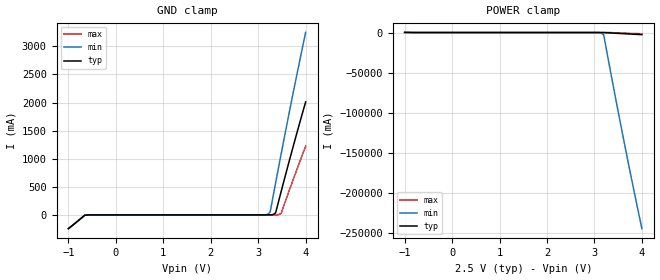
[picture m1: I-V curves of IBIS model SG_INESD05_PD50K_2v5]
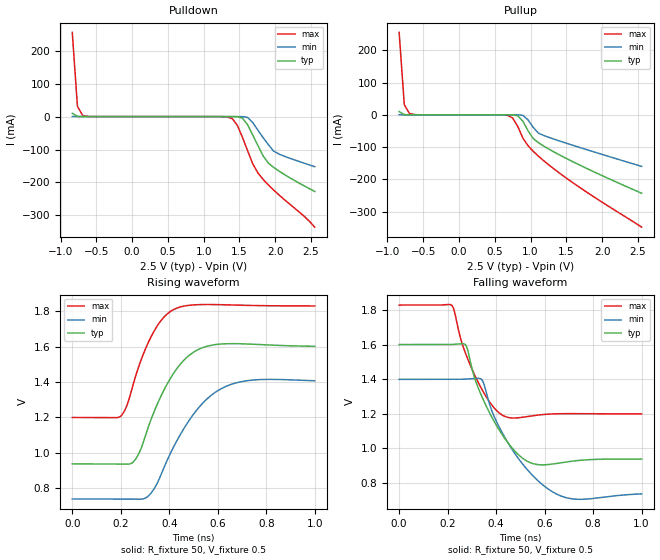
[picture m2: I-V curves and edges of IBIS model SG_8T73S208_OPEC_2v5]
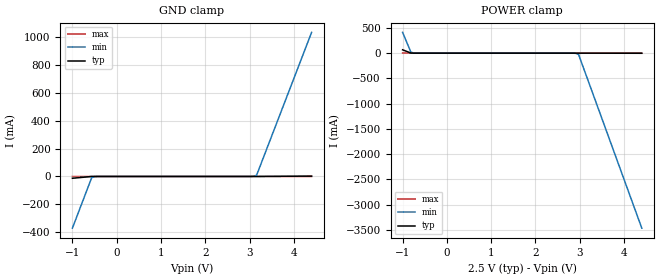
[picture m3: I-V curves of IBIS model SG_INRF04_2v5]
|   This file is an IBIS representation of the   |
|   Integrated Device Technology Inc   |
|   IDT8T732S208I-01   |
|   2.5V DIFFERENTIAL LVPECL CLOCK DIVIDER AND FANOUT BUFFER   |
[IBIS Ver]   4.1
[File name]   8t73s208i_01.ibs
[File Rev]   1.0
[Date]   14 APR 2015
[Source]   Originated at Integrated Device Technology, Inc.
[Disclaimer]
IDT hereby grants the user of this IBIS model a non-exclusive,
nontransferable license to use this IBIS model under the following terms.
Before using this IBIS model, the user should read this license.
If the user does not accept these terms,  the IBIS model should be
returned to IDT within 30 days.
   The user is granted this license only to use the IBIS model and
is not granted rights to sell, load, rent, lease or license the IBIS
model in whole or in part, or in modified form to anyone other than
user. User may modify the IBIS model to suit its specific
applications but rights to derivative works and such modifications
shall belong to IDT.
   This IBIS model is provided on an "AS IS" basis and IDT makes
absolutely no warranty with respect to the information contained
herein. IDT DISCLAIMS AND CUSTOMER WAIVES ALL WARRANTIES, EXPRESS
OR IMPLIED, INCLUDING WARRANTIES OF MERCHANTABILITY OR FITNESS FOR
A PARTICULAR PURPOSE. The entire risk as to quality and performance
is with the Customer. ACCORDINGLY, IN NO EVENT SHALL THE COMPANY BE
LIABLE FOR ANY DAMAGES, WHETHER IN CONTRACT OR TORT,INCLUDING ANY
LOST PROFITS OR OTHER INCIDENTAL, CONSEQUENTIAL, EXEMPLARY, OR
PUNITIVE DAMAGES ARISING OUT OF THE USE OR APPLICATION OF THE IBIS
model provided in this package. Further, IDT reserves the right to
make changes without notice to any product herein to improve
reliability, function, or design. IDT does not convey any license
under patent rights or any other intellectual property rights,
including those of third parties.
   IDT is not obligated to provide maintenance or support
for the licensed IBIS model.
[Copyright]   Copyright 2015 by IDT Inc.
[Component]   IDT8T73S208-01NGLI
[Manufacturer] Integrated Device Technology, Inc.
[Package]
|QFN 32
|lead + wire   typ   min   max
R_pkg   148.525m   92.309m   189.241m
L_pkg   1.318n   1.032n   1.634n
C_pkg   203.71f   184.14f   234.70f
[Pin] signal_name  model_name   R_pin   L_pin   C_pin
1   ADR1   SG_INESD05_PD50K   179.610m   1.461n   191.255f
2   VEE   GND   161.763m   1.447n   217.440f
3   Q0   SG_8T73S208_OPEC   133.456m   1.141n   193.994f
4   nQ0   SG_8T73S208_OPEC   121.044m   1.074n   185.939f
5   Q1   SG_8T73S208_OPEC   121.059m   1.076n   185.852f
6   nQ1   SG_8T73S208_OPEC   133.102m   1.147n   191.453f
7   VEE   GND   155.227m   1.389n   208.655f
8   VCCO   POWER   92.957m   1.034n   234.700f
9   Q2   SG_8T73S208_OPEC   189.241m   1.628n   200.299f
10   nQ2   SG_8T73S208_OPEC   162.649m   1.454n   218.396f
11   Q3   SG_8T73S208_OPEC   148.929m   1.333n   206.721f
12   nQ3   SG_8T73S208_OPEC   141.884m   1.269n   201.683f
13   Q4   SG_8T73S208_OPEC   140.676m   1.266n   201.115f
14   nQ4   SG_8T73S208_OPEC   147.702m   1.330n   206.004f
15   Q5   SG_8T73S208_OPEC   162.346m   1.447n   217.794f
16   nQ5   SG_8T73S208_OPEC   187.699m   1.617n   199.589f
17   VCCO   POWER   92.309m   1.032n   233.375f
18   VEE   GND   160.583m   1.439n   216.539f
19   Q6   SG_8T73S208_OPEC   130.493m   1.132n   190.219f
20   nQ6   SG_8T73S208_OPEC   119.346m   1.058n   184.145f
21   Q7   SG_8T73S208_OPEC   119.470m   1.058n   184.836f
22   nQ7   SG_8T73S208_OPEC   131.938m   1.123n   192.881f
23   VEE   GND   154.094m   1.380n   207.790f
24   FSEL0   SG_INESD05_PD50K   178.400m   1.450n   190.311f
25   FSEL1   SG_INESD05_PD50K   188.238m   1.619n   199.880f
26   IN   SG_INRF04   162.205m   1.453n   218.726f
27   VT   NC   148.673m   1.335n   206.818f
28   nIN   SG_INRF04   142.492m   1.275n   201.850f
29   VCC   POWER   143.017m   1.278n   202.447f
30   SDA   SG_I2C_DATAOUT02   149.682m   1.341n   207.211f
31   SCL   SG_I2C_SCLOCK03   163.397m   1.462n   219.637f
32   ADR0   SG_INESD05_PD50K   189.125m   1.634n   201.172f
[Diff Pin]  inv_pin   vdiff   tdelay_typ   tdelay_min   tdelay_max
3   4   NA   0   0   0
5   6   NA   0   0   0
9   10   NA   0   0   0
11   12   NA   0   0   0
13   14   NA   0   0   0
15   16   NA   0   0   0
19   20   NA   0   0   0
21   22   NA   0   0   0
26   28   0.15   NA   NA   NA
[Series Pin Mapping] Pin_2   model_name   function_table_group
26   28   ODT_100
[Model Selector] SG_INESD05_PD50K
SG_INESD05_PD50K_2v5  Buffer selection for 2v5
SG_INESD05_PD50K_3v3  Buffer selection for 3v3
[Model Selector] SG_8T73S208_OPEC
SG_8T73S208_OPEC_2v5  Buffer selection for 2v5
SG_8T73S208_OPEC_3v3  Buffer selection for 3v3
[Model Selector] SG_INRF04
SG_INRF04_2v5  Buffer selection for 2v5
SG_INRF04_3v3  Buffer selection for 3v3
[Model Selector] SG_I2C_DATAOUT02
SG_I2C_DATAOUT02_2v5  Buffer selection for 2v5
SG_I2C_DATAOUT02_3v3  Buffer selection for 3v3
[Model Selector] SG_I2C_SCLOCK03
SG_I2C_SCLOCK03_2v5  Buffer selection for 2v5
SG_I2C_SCLOCK03_3v3  Buffer selection for 3v3
[Model]   ODT_100
Model_type  Series
Polarity   Non-Inverting
|   typ   min   max
C_comp   0pF   0pF   0pF
|   typ   min   max
[Voltage Range]   3.3V   3.135V   3.465V
[R Series]   100ohm   80ohm   120ohm
| Models and submodels in the file (11): ODT_100 (Series), SG_INESD05_PD50K_2v5 (Input), SG_8T73S208_OPEC_2v5 (Output_ECL), SG_INRF04_2v5 (Input), SG_I2C_DATAOUT02_2v5 (Input), SG_I2C_SCLOCK03_2v5 (Input), SG_INESD05_PD50K_3v3 (Input), SG_8T73S208_OPEC_3v3 (Output_ECL), SG_INRF04_3v3 (Input), SG_I2C_DATAOUT02_3v3 (Input), SG_I2C_SCLOCK03_3v3 (Input)
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[Model] SG_INESD05_PD50K_2v5
Model_type   Input
Polarity   Non-Inverting
Vinl = 0.7V
Vinh = 1.7V
|   typ   min   max
C_comp   2pF   1.5pF   2.5pF
|   typ   min   max
[Voltage range]   2.5V   2.375V   2.625V
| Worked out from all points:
|   GND clamp passes 1 mA (typ) near -0.58 V on its own axis
|   POWER clamp passes 1 mA (typ) near -0.76 V on its own axis
[GND_clamp]
|Voltage   I (typ)   I (min)   I (max)
-999mV    -244.8mA   -244.8mA   -244.8mA
-654.2mV  -6.145mA   -6.145mA   -6.145mA
-596.8mV  -1.247mA   -1.247mA   -1.247mA
3.196V    197uA      6.481mA    69.73uA
3.253V    701.9uA    51.67mA    91.7uA
3.31V     4.516mA    312.6mA    170.5uA
3.368V    36.44mA    571mA      537.5uA
3.483V    411.8mA    1.08A      25.29mA
3.713V    1.14A      2.068A     570.6mA
4V        2.011A     3.248A     1.222A
[Power_clamp]
|Voltage   I (typ)   I (min)   I (max)
-999mV    170.5mA    170.5mA    170.5mA
3.081V    -874.7uA   -37.46mA   -65.82uA
3.138V    -3.712mA   -330.8mA   -230uA
3.196V    -25.84mA   -3.028A    -710.8uA
3.368V    -616.5mA   -57.72A    -152.9mA
3.598V    -1.377A    -128.1A    -679.2mA
3.77V     -1.927A    -179.1A    -1.06A
4V        -2.636A    -244.7A    -1.551A
[Model] SG_8T73S208_OPEC_2v5
Model_type   Output_ECL
Polarity   Non-Inverting
|   typ   min   max
C_comp   2pF   1.5pF   2.5pF
Vmeas = 1.27V
Rref = 50
Cref = 0
Vref = 0.5V
|   typ   min   max
[Voltage range]   2.5V   2.375V   2.625V
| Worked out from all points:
|   rising waveform, R_fixture 50, V_fixture 0.5: 20-80 % time 132ps typ, 168ps min, 105ps max; typ from 0.935 V to 1.6 V
|   falling waveform, R_fixture 50, V_fixture 0.5: 20-80 % time 130ps typ, 163ps min, 106ps max; typ from 1.6 V to 0.936 V
[Pulldown]
|Voltage   I (typ)   I (min)   I (max)
|Note, modeling breaks down at 250mA and above.  This is well beyond the functional   |
|operating range of the device.  Should this scenario occur, catastrophic failure and   |
|possible damage to the device and/or board is of higher concern than the I-V curve   |
|behavior.  The IBIS checker will flag currents in excess of 10A with warnings.  Lines   |
|with currents in excess of 0.35 A have been commented out.  The points still remain|
|available to the user if the user desires to use them.   |
|-2.40000e+00   2.40058e+08   3.18314e+08   1.70330e+08
|-2.30000e+00   2.17517e+08   2.89489e+08   1.53450e+08
|-2.20000e+00   1.94976e+08   2.60664e+08   1.36571e+08
|-2.10000e+00   1.72434e+08   2.31839e+08   1.19691e+08
|-2.00000e+00   1.49893e+08   2.03013e+08   1.02811e+08
|-1.99000e+00   1.47639e+08   2.00131e+08   1.01123e+08
|-1.91789e+00   1.31385e+08   1.79344e+08   8.89513e+07
|-1.84578e+00   1.15130e+08   1.58558e+08   7.67792e+07
|-1.77367e+00   9.88755e+07   1.37772e+08   6.46072e+07
|-1.70156e+00   8.26209e+07   1.16986e+08   5.24351e+07
|-1.62944e+00   6.63663e+07   9.61996e+07   4.02630e+07
|-1.55733e+00   5.01117e+07   7.54133e+07   2.80910e+07
|-1.48522e+00   3.38571e+07   5.46271e+07   1.59189e+07
|-1.41311e+00   1.76025e+07   3.38409e+07   4.06873e+06
|-1.34100e+00   2.68882e+06   1.30547e+07   4.97358e+05
|-1.26889e+00   1.62424e+05   5.60643e+05   6.08111e+04
|-1.19678e+00   9.82536e+03   1.55006e+04   7.44651e+03
|-1.12467e+00   6.03162e+02   4.37674e+02   9.19844e+02
|-1.05256e+00   4.08696e+01   1.46783e+01   1.18373e+02
|-9.80444e-01   2.72626e+00   4.11433e-01   1.67167e+01
|-9.08333e-01   1.64665e-01   1.13631e-02   2.09236e+00
-836.2mV  9.946mA    313.8uA    255.8mA
-764.1mV  600.7uA    8.668uA    31.26mA
-692mV    36.28uA    239.4nA    3.821mA
1.399V    -23.93uA   -81.46nA   -6.063mA
1.471V    -371.6uA   -2.797uA   -26.61mA
1.543V    -4.74mA    -95.28uA   -63.33mA
1.616V    -25.22mA   -2.607mA   -104.3mA
1.688V    -56.51mA   -18.58mA   -143.8mA
1.76V     -88.62mA   -41.74mA   -171.4mA
1.832V    -119.4mA   -64.05mA   -190.7mA
1.976V    -153.8mA   -104.3mA   -222.5mA
2.553V    -227.4mA   -152mA     -335.5mA
| 2.62511e+00   -2.35788e-01   -1.57199e-01   -3.55079e-01
| 2.69722e+00   -2.44484e-01   -1.62478e-01   -3.76294e-01
| 2.76933e+00   -2.54060e-01   -1.67881e-01   -3.98352e-01
| 2.84144e+00   -2.64769e-01   -1.73383e-01   -4.20357e-01
| 2.91356e+00   -2.76399e-01   -1.79146e-01   -4.42244e-01
| 2.98567e+00   -2.88756e-01   -1.85542e-01   -4.64335e-01
| 3.05778e+00   -3.01671e-01   -1.92630e-01   -4.83732e-01
| 3.12989e+00   -3.14773e-01   -2.00258e-01   -5.01249e-01
| 3.20200e+00   -3.28189e-01   -2.08432e-01   -5.18585e-01
| 3.27411e+00   -3.42273e-01   -2.18697e-01   -5.37304e-01
| 3.34622e+00   -3.64261e-01   -2.55817e-01   -5.66211e-01
| 3.41833e+00   -4.09420e-01   -3.05414e-01   -6.08363e-01
| 3.49044e+00   -4.54655e-01   -3.54748e-01   -6.50575e-01
| 3.56256e+00   -4.99420e-01   -4.03513e-01   -6.92819e-01
| 3.63467e+00   -5.44118e-01   -4.52081e-01   -7.35068e-01
| 3.70678e+00   -5.88861e-01   -5.00706e-01   -7.77241e-01
| 3.77889e+00   -6.33554e-01   -5.49415e-01   -8.19100e-01
| 3.85100e+00   -6.78004e-01   -5.98203e-01   -8.60639e-01
| 3.92311e+00   -7.21963e-01   -6.47066e-01   -9.01982e-01
| 3.99522e+00   -7.65389e-01   -6.95996e-01   -9.43201e-01
| 4.06733e+00   -8.08562e-01   -7.44993e-01   -9.84333e-01
| 4.13944e+00   -8.51732e-01   -7.94061e-01   -1.02539e+00
| 4.21156e+00   -8.94966e-01   -8.43201e-01   -1.06639e+00
| 4.28367e+00   -9.38253e-01   -8.92407e-01   -1.10739e+00
| 4.35578e+00   -9.81577e-01   -9.41676e-01   -1.14879e+00
| 4.42789e+00   -1.02499e+00   -9.91033e-01   -1.19324e+00
| 4.50000e+00   -1.06928e+00   -1.04102e+00   -1.23986e+00
| 4.51000e+00   -1.07571e+00   -1.04813e+00   -1.24627e+00
| 4.60800e+00   -1.14301e+00   -1.12225e+00   -1.30851e+00
| 4.70600e+00   -1.21072e+00   -1.19824e+00   -1.37003e+00
| 4.80400e+00   -1.27948e+00   -1.27431e+00   -1.43183e+00
| 4.90200e+00   -1.35101e+00   -1.35037e+00   -1.49633e+00
| 5.00000e+00   -1.42381e+00   -1.42638e+00   -1.56424e+00
[Pullup]
|Voltage   I (typ)   I (min)   I (max)
|Note, modeling breaks down at 250mA and above.  This is well beyond the functional   |
|operating range of the device.  Should this scenario occur, catastrophic failure and   |
|possible damage to the device and/or board is of higher concern than the I-V curve   |
|behavior.  The IBIS checker will flag currents in excess of 10A with warnings.  Lines   |
|with currents in excess of 0.35 A have been commented out.  The points still remain|
|available to the user if the user desires to use them.   |
|-2.40000e+00   2.40058e+08   3.18314e+08   1.70330e+08
|-2.30000e+00   2.17517e+08   2.89489e+08   1.53450e+08
|-2.20000e+00   1.94976e+08   2.60664e+08   1.36571e+08
|-2.10000e+00   1.72434e+08   2.31839e+08   1.19691e+08
|-2.00000e+00   1.49893e+08   2.03013e+08   1.02811e+08
|-1.99000e+00   1.47639e+08   2.00131e+08   1.01123e+08
|-1.91789e+00   1.31385e+08   1.79344e+08   8.89513e+07
|-1.84578e+00   1.15130e+08   1.58558e+08   7.67792e+07
|-1.77367e+00   9.88755e+07   1.37772e+08   6.46072e+07
|-1.70156e+00   8.26209e+07   1.16986e+08   5.24351e+07
|-1.62944e+00   6.63663e+07   9.61996e+07   4.02630e+07
|-1.55733e+00   5.01117e+07   7.54133e+07   2.80910e+07
|-1.48522e+00   3.38571e+07   5.46271e+07   1.59189e+07
|-1.41311e+00   1.76025e+07   3.38409e+07   4.06873e+06
|-1.34100e+00   2.68882e+06   1.30547e+07   4.97358e+05
|-1.26889e+00   1.62424e+05   5.60643e+05   6.08111e+04
|-1.19678e+00   9.82536e+03   1.55006e+04   7.44651e+03
|-1.12467e+00   6.03162e+02   4.37674e+02   9.19844e+02
|-1.05256e+00   4.08696e+01   1.46783e+01   1.18373e+02
|-9.80444e-01   2.72626e+00   4.11433e-01   1.67167e+01
|-9.08333e-01   1.64665e-01   1.13631e-02   2.09236e+00
-836.2mV  9.946mA    313.8uA    255.8mA
-764.1mV  600.7uA    8.668uA    31.26mA
-692mV    36.28uA    239.4nA    3.821mA
678.1mV   -14.48uA   -54.93nA   -1.577mA
750.2mV   -226.4uA   -1.885uA   -9.926mA
822.3mV   -3.108mA   -64.41uA   -36.27mA
894.4mV   -20.23mA   -1.876mA   -72.78mA
1.039V    -73.94mA   -39.15mA   -113.4mA
1.111V    -86.46mA   -56.96mA   -128.4mA
1.183V    -96.82mA   -63.97mA   -142.2mA
1.688V    -155.9mA   -101.3mA   -225.3mA
2.553V    -243.3mA   -160mA     -348.5mA
| 2.62511e+00   -2.50387e-01   -1.64771e-01   -3.59518e-01
| 2.69722e+00   -2.57594e-01   -1.69555e-01   -3.72316e-01
| 2.76933e+00   -2.64885e-01   -1.74366e-01   -3.87671e-01
| 2.84144e+00   -2.72208e-01   -1.79242e-01   -4.05741e-01
| 2.91356e+00   -2.79574e-01   -1.84271e-01   -4.25992e-01
| 2.98567e+00   -2.87321e-01   -1.89722e-01   -4.47114e-01
| 3.05778e+00   -2.96533e-01   -1.95679e-01   -4.68617e-01
| 3.12989e+00   -3.07573e-01   -2.02058e-01   -4.90289e-01
| 3.20200e+00   -3.19975e-01   -2.08904e-01   -5.11805e-01
| 3.27411e+00   -3.34016e-01   -2.18132e-01   -5.33959e-01
| 3.34622e+00   -3.56179e-01   -2.54416e-01   -5.65575e-01
| 3.41833e+00   -4.02130e-01   -3.03378e-01   -6.09689e-01
| 3.49044e+00   -4.48787e-01   -3.52496e-01   -6.52787e-01
| 3.56256e+00   -4.95341e-01   -4.01686e-01   -6.95001e-01
| 3.63467e+00   -5.41211e-01   -4.50852e-01   -7.36639e-01
| 3.70678e+00   -5.85960e-01   -4.99624e-01   -7.77908e-01
| 3.77889e+00   -6.30161e-01   -5.48368e-01   -8.18937e-01
| 3.85100e+00   -6.74093e-01   -5.97153e-01   -8.59793e-01
| 3.92311e+00   -7.17871e-01   -6.45989e-01   -9.00510e-01
| 3.99522e+00   -7.61550e-01   -6.94878e-01   -9.41084e-01
| 4.06733e+00   -8.05163e-01   -7.43823e-01   -9.81499e-01
| 4.13944e+00   -8.48736e-01   -7.92832e-01   -1.02174e+00
| 4.21156e+00   -8.92288e-01   -8.41909e-01   -1.06180e+00
| 4.28367e+00   -9.35825e-01   -8.91049e-01   -1.10177e+00
| 4.35578e+00   -9.79351e-01   -9.40247e-01   -1.14226e+00
| 4.42789e+00   -1.02293e+00   -9.89545e-01   -1.18633e+00
| 4.50000e+00   -1.06742e+00   -1.03964e+00   -1.23277e+00
| 4.51000e+00   -1.07388e+00   -1.04679e+00   -1.23919e+00
| 4.60800e+00   -1.14138e+00   -1.12122e+00   -1.30175e+00
| 4.70600e+00   -1.20927e+00   -1.19727e+00   -1.36399e+00
| 4.80400e+00   -1.27873e+00   -1.27338e+00   -1.42722e+00
| 4.90200e+00   -1.35081e+00   -1.34953e+00   -1.49362e+00
| 5.00000e+00   -1.42383e+00   -1.42570e+00   -1.56248e+00
[Ramp]
|   typ   min   max
dV/dt_r   0.409/0.137n   0.407/0.172n   0.384/0.108n
dV/dt_f   0.421/0.142n   0.421/0.178n   0.395/0.113n
R_load =   50.0000
[Rising Waveform]
R_fixture = 50
V_fixture = 0.5   | VCC_typ - 2V
V_fixture_max = 0.625   | VCC_max - 2V
V_fixture_min = 0.375   | VCC_min - 2V
C_fixture = 0.0p
| Time   typ   min   max
0s        935.3mV    736.8mV    1.198V
195.2ps   934.5mV    736.6mV    1.202V
223.2ps   933.5mV    736.5mV    1.259V
250.2ps   944.8mV    735.6mV    1.381V
281.3ps   1.014V     735.3mV    1.515V
327.3ps   1.196V     774.6mV    1.662V
423.4ps   1.46V      1.046V     1.813V
526.5ps   1.588V     1.262V     1.838V
630.6ps   1.616V     1.373V     1.836V
1ns       1.601V     1.406V     1.83V
[Falling Waveform]
R_fixture = 50
V_fixture = 0.5   | VCC_typ - 2V
V_fixture_max = 0.625   | VCC_max - 2V
V_fixture_min = 0.375   | VCC_min - 2V
C_fixture = 0.0p
| Time   typ   min   max
0s        1.601V     1.399V     1.83V
216.2ps   1.601V     1.399V     1.829V
272.3ps   1.601V     1.4V       1.555V
342.3ps   1.295V     1.394V     1.338V
384.4ps   1.174V     1.208V     1.246V
433.4ps   1.06V      1.068V     1.185V
536.5ps   917.8mV    861.8mV    1.185V
662.7ps   913.8mV    724.5mV    1.199V
752.8ps   929.7mV    702.7mV    1.2V
1ns       935.9mV    734.2mV    1.198V
[Model] SG_INRF04_2v5
Model_type   Input
Polarity   Non-Inverting
Vinl = 0.7V
Vinh = 1.7V
|   typ   min   max
C_comp   2pF   1.5pF   2.5pF
|   typ   min   max
[Voltage range]   2.5V   2.375V   2.625V
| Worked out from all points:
|   GND clamp passes 1 mA (typ) near -0.59 V on its own axis
|   POWER clamp passes 1 mA (typ) near -0.77 V on its own axis
[GND_clamp]
|Voltage   I (typ)   I (min)   I (max)
-999mV    -12.93mA   -371.3mA   -72.72uA
-564.6mV  -301.6uA   -9.176mA   -500.3nA
-502.5mV  -33.51uA   -1.674mA   -23.2nA
2.973V    11.79nA    53.54uA    48.4pA
3.097V    1.338uA    1.663mA    283.7pA
3.159V    14.74uA    9.108mA    753.2pA
4.4V      2.639mA    1.035A     64.91nA
[Power_clamp]
|Voltage   I (typ)   I (min)   I (max)
-999mV    66.35mA    411.4mA    4.504mA
-812.8mV  2.746mA    21.64mA    126.7uA
-750.8mV  393.7uA    3.585mA    6.636uA
2.787V    -8.042nA   -146.4uA   -27.5pA
2.911V    -969.4nA   -4.038mA   -30.98pA
2.973V    -10.73uA   -24.72mA   -42.86pA
4.4V      -2.275mA   -3.463A    -5.326nA
